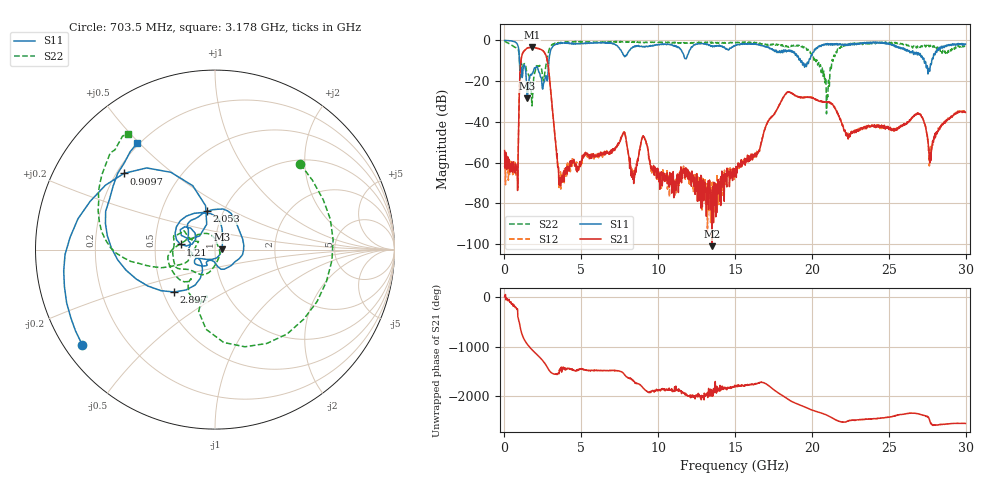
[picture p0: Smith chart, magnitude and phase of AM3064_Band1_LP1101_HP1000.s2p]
# Hz S DB R 50.0
!freq dBS11 angS11 dBS21 angS21 dBS12 angS12 dBS22 angS22
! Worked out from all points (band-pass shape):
!   1600 points, 10 MHz to 29.98 GHz, reference 50 ohm
!   highest |S21| = -3.37 dB at 1.791 GHz (marker M1); lowest = -101.1 dB at 13.51 GHz (marker M2)
!   |S21| within 3 dB of the highest: 1.178 GHz to 2.631 GHz (1.453 GHz wide, 76.3 % of centre)
!   lowest |S11| = -28.4 dB at 1.472 GHz (marker M3), VSWR 1.08, Z = 53.9 + j0.138 ohm
!   |S11| at or under -10 dB: 974 MHz to 2.893 GHz (1.919 GHz wide, 99.2 % of centre); 19.26 GHz to 19.8 GHz (543.8 MHz wide, 2.78 % of centre); 27.3 GHz to 27.79 GHz (494 MHz wide, 1.79 % of centre)
!   |S22| runs from -36.1 to -0.3 dB; largest |S21 - S12| = 0.0098
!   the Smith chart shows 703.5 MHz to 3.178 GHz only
!   S11 on the Smith chart (normalised r, x): 703.5 MHz: 0.05, -0.32; 909.7 MHz: 0.23, +0.35; 1.21 GHz: 0.68, +0.04; 2.053 GHz: 0.84, +0.38; 2.897 GHz: 0.57, -0.30; 3.178 GHz: 0.19, +0.49
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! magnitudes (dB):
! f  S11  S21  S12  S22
! 10 MHz  0.0  -54.1  -62.1  -0.3
! 703.5 MHz  -0.8  -65.2  -65.6  -3.4
! 909.7 MHz  -3.6  -47.1  -47.2  -4.9
! 1.21 GHz  -14.2  -5.9  -5.9  -12.6
! 1.472 GHz  -28.4  -3.9  -3.8  -15.5
! 1.791 GHz  -16.4  -3.4  -3.4  -32.2
! 2.053 GHz  -13.2  -3.8  -3.8  -13.1
! 2.897 GHz  -9.7  -16.0  -15.9  -4.7
! 3.178 GHz  -2.7  -38.5  -38.7  -1.9
! 3.665 GHz  -1.5  -69.3  -73.0  -1.0
! 5.015 GHz  -1.5  -59.1  -58.9  -0.6
! 7.751 GHz  -7.4  -45.2  -45.0  -0.7
! 8.388 GHz  -3.3  -65.5  -66.0  -1.0
! 9.063 GHz  -3.0  -47.5  -47.5  -1.0
! 10 GHz  -2.1  -64.4  -65.1  -0.9
! 13.51 GHz  -2.7  -101.1  -74.5  -1.0
! 15 GHz  -2.6  -64.3  -65.7  -1.3
! 19.99 GHz  -7.5  -28.2  -28.1  -6.8
! 20.98 GHz  -1.7  -30.4  -30.2  -25.9
! 25 GHz  -1.4  -43.4  -42.7  -1.3
! 27.71 GHz  -11.6  -55.2  -55.9  -2.5
! 29.98 GHz  -1.8  -35.4  -35.2  -2.9
